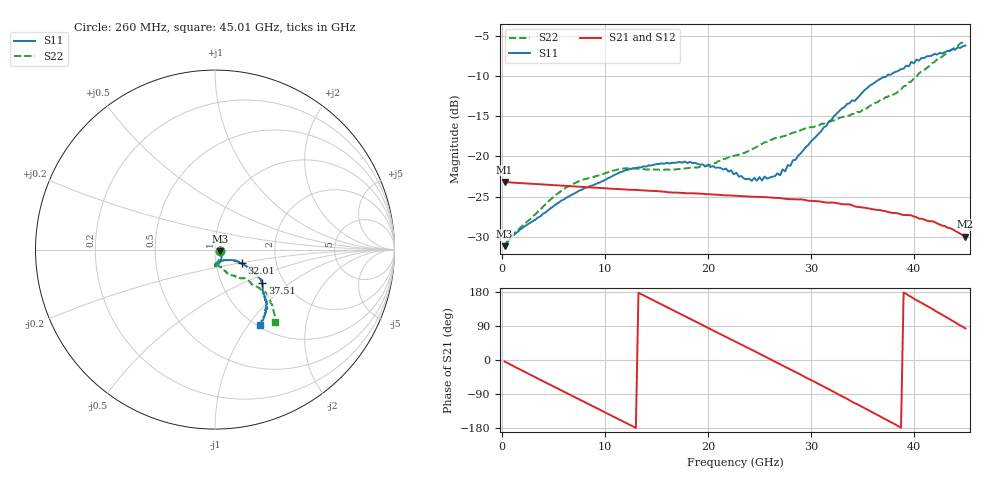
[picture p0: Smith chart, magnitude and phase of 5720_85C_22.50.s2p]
! Device:  ADRF5720
! Description: 0.5dB LSB GaAs MMIC 6-bit Digital Attenuator
! Frequency:  0.000009 -  40 GHz
! Ports:
!	RF1	= Port 1
!	RF2	= Port 2
! Vdd:  3.3 Volt
! Vss:  -3.3 Volt
! Control:  0/3.3 Volt
! State:  22.50 dB attenuation
! Data:  The device was measured using G-S-G Probes on a matrix board.
!  Data was collected using an calibrated 4 port network analyzer.
!  The reference plane for this measurement is at the launchers.
! Note:  Analog Devices supplies this data as a sample of measured data
!  for this product.  Your particular data for this product may vary.
!  Data was taken at 85 degrees C.
!  Analog Devices reserves the right to change this data at anytime.
# GHZ S DB R 45.0
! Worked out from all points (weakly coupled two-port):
!   180 points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, 260 MHz to 45.01 GHz, reference 45 ohm
!   highest |S21| = -23.19 dB at 260 MHz (marker M1); lowest = -30.0 dB at 45.01 GHz (marker M2)
!   lowest |S11| = -31.2 dB at 260 MHz (marker M3), VSWR 1.06, Z = 47.4 - j0.762 ohm
!   |S11| at or under -10 dB: start of sweep to 37.37 GHz
!   |S22| runs from -31.1 to -5.6 dB; largest |S21 - S12| = 0.00035
!   S11 on the Smith chart (normalised r, x): 260 MHz: 1.05, -0.02; 32.01 GHz: 1.33, -0.21; 37.51 GHz: 1.55, -0.64; 45.01 GHz: 1.03, -1.14
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0.26  -31.17 -16.9  -23.19 -3.9  -23.19 -3.8  -31.08 -17.6
1.76  -29.12 -6.7  -23.32 -25.1  -23.30 -25.0  -28.90 -18.0
5.01  -26.19 -39.7  -23.57 -69.9  -23.55 -69.8  -25.04 -61.6
7.76  -24.16 -55.8  -23.79 -107.5  -23.77 -107.4  -22.96 -78.1
11.51  -21.97 -73.5  -24.08 -158.6  -24.07 -158.5  -21.55 -91.8
15.26  -20.96 -84.8  -24.34 149.8  -24.33 149.9  -21.65 -93.4
18.26  -20.69 -90.0  -24.59 109.0  -24.57 109.1  -21.42 -87.0
22.76  -22.03 -83.9  -24.91 47.3  -24.89 47.5  -19.86 -72.6
24.26  -23.04 -76.0  -25.02 26.9  -25.00 27.1  -19.14 -69.3
27.01  -22.36 -50.0  -25.18 -11.2  -25.17 -11.0  -17.61 -64.1
27.26  -21.61 -46.2  -25.24 -14.8  -25.22 -14.6  -17.51 -64.5
27.51  -21.87 -45.4  -25.27 -18.1  -25.26 -17.9  -17.45 -63.5
27.76  -21.08 -41.8  -25.29 -21.5  -25.27 -21.2  -17.25 -64.2
28.01  -21.19 -42.1  -25.33 -25.0  -25.31 -24.8  -17.20 -63.5
30.26  -17.84 -30.0  -25.54 -56.2  -25.52 -56.0  -16.38 -61.5
32.01  -15.46 -27.1  -25.74 -80.8  -25.72 -80.6  -15.61 -58.4
35.76  -11.16 -31.7  -26.51 -134.8  -26.48 -134.6  -13.68 -49.6
37.51  -9.83 -35.2  -26.93 -160.4  -26.91 -160.0  -12.55 -43.2
37.76  -9.84 -35.6  -27.00 -163.9  -26.99 -163.5  -12.35 -43.3
41.51  -7.53 -47.3  -28.07 139.3  -28.05 139.7  -8.77 -40.1
43.51  -6.89 -51.5  -28.93 107.7  -28.90 108.0  -6.82 -45.1
45.01  -6.20 -59.4  -29.97 83.3  -29.94 83.7  -5.58 -50.4
